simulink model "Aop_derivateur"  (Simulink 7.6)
settings: Solver=ode15s  StartTime=0.0  StopTime=1.4  RelTol=1e-3
InitFcn:
  | close all, clear all, clc
StopFcn:
  | close all, clc
  | load es.mat
  | plotyy(x(1,:),x(2,:),x(1,:),x(3,:))
  | title('montage dérivateur')
  | xlabel('temps')
  | grid
libraries: fl_lib x8, nesl_utility x3, simulink x1

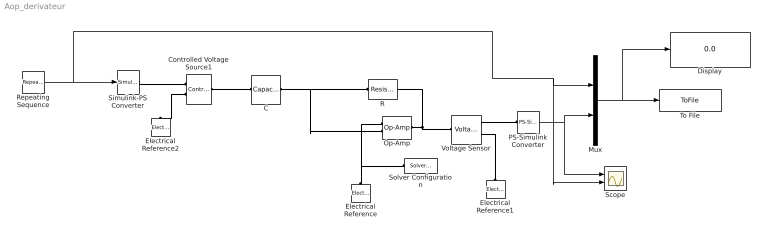
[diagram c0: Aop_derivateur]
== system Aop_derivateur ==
  C : fl_lib/Electrical/Electrical Elements/Capacitor  DialogController=NetworkEngine.DynNeDlgSource  SystemSampleTime=-1  c=100e-9 F  v0=0 V  r=1e-6 Ohm  g=0 1/Ohm  i_Log=off  v_Log=off  vc_Log=off  LocalVarNames=|current|voltage|power  LocalVarDescs=|Capacitor current (A)|Voltage across capacitor (V)|Power (W)  LocalVarLogging=[0 0 0]
  Controlled Voltage Source1 : fl_lib/Electrical/Electrical Sources/Controlled Voltage Source  DialogController=NetworkEngine.DynNeDlgSource  SystemSampleTime=-1  i_Log=off  v_Log=off  LocalVarNames=|current|voltage|power  LocalVarDescs=|Current (A)|Voltage (V)|Power (W)  LocalVarLogging=[0 0 0]
  Display : Display
  Electrical Reference : fl_lib/Electrical/Electrical Elements/Electrical Reference  DialogController=NetworkEngine.DynNeDlgSource  SystemSampleTime=-1  i_Log=off  LocalVarNames=|i  LocalVarDescs=|i  LocalVarLogging=[]
  Electrical Reference1 : fl_lib/Electrical/Electrical Elements/Electrical Reference  DialogController=NetworkEngine.DynNeDlgSource  SystemSampleTime=-1  i_Log=off  LocalVarNames=|i  LocalVarDescs=|i  LocalVarLogging=[]
  Electrical Reference2 : fl_lib/Electrical/Electrical Elements/Electrical Reference  DialogController=NetworkEngine.DynNeDlgSource  SystemSampleTime=-1  i_Log=off  LocalVarNames=|i  LocalVarDescs=|i  LocalVarLogging=[]
  Mux : Mux  Inputs=2
  Op-Amp : fl_lib/Electrical/Electrical Elements/Op-Amp  DialogController=NetworkEngine.DynNeDlgSource  SystemSampleTime=-1  i1_Log=off  v1_Log=off  outI_Log=off  LocalVarNames=|i1|v1|outI  LocalVarDescs=|i1|v1|outI  LocalVarLogging=[]
  PS-Simulink Converter : nesl_utility/PS-Simulink Converter  DialogController=NetworkEngine.DynNeUtilDlgSource  SystemSampleTime=-1  PhysicalDomain=network_engine_domain  LeftPortType=input  RightPortType=output  SubClassName=ps_output  Unit=1  AffineConversion=off
  R : fl_lib/Electrical/Electrical Elements/Resistor  DialogController=NetworkEngine.DynNeDlgSource  SystemSampleTime=-1  R=10e3 Ohm  i_Log=off  v_Log=off  LocalVarNames=|current|voltage|power  LocalVarDescs=|Resistor current (A)|Voltage across resistor (V)|Power (W)  LocalVarLogging=[0 0 0]
  Repeating Sequence : simulink/Sources/Repeating Sequence  SystemSampleTime=-1  rep_seq_t="[0  0.7 1.4 2.1 2.8 3.5 4.2 4.9]"  rep_seq_y="[0  0.1  0 .1 0  0.1  0 .1]"
  Scope : Scope  NumInputPorts=2
  Simulink-PS Converter : nesl_utility/Simulink-PS Converter  DialogController=NetworkEngine.DynNeUtilDlgSource  SystemSampleTime=-1  PhysicalDomain=network_engine_domain  LeftPortType=input  RightPortType=output  SubClassName=ps_input  Unit=1  AffineConversion=off  InputFilterTimeConstant=.001  UdotUserProvided=0
  Solver Configuration : nesl_utility/Solver Configuration  DialogController=NetworkEngine.DynNeUtilDlgSource  SystemSampleTime=-1  PhysicalDomain=network_engine_domain  LeftPortType=input  RightPortType=generic  SubClassName=solver  Accelerate=off  Profile=off  ResidualTolerance=1e-9  MaxNonlinIter=12  MaxModeIter=2  DoFixedCost=off  UseLocalSampling=off  DoDC=off  LinearAlgebra=Sparse  LocalSolverSampleTime=.001  LocalSolverChoice=NE_BACKWARD_EULER_ADVANCER  UseLocalSolver=off
  To File : ToFile  Filename=es.mat  MatrixName=x
  Voltage Sensor : fl_lib/Electrical/Electrical Sensors/Voltage Sensor  DialogController=NetworkEngine.DynNeDlgSource  SystemSampleTime=-1  i1_Log=off  v1_Log=off  LocalVarNames=|i1|v1  LocalVarDescs=|i1|v1  LocalVarLogging=[]
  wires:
  PS-Simulink Converter/1 -> Mux/2, Scope/1
  Mux/1 -> To File/1, Display/1
  Repeating Sequence/1 -> Simulink-PS Converter/1, Mux/1, Scope/2
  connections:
  Electrical Reference/LConn1 -- Op-Amp/LConn1 -- Solver Configuration/RConn1
  C/RConn1 -- R/LConn1 -- Op-Amp/LConn2
  Electrical Reference1/LConn1 -- Voltage Sensor/RConn2
  Voltage Sensor/RConn1 -- PS-Simulink Converter/LConn1
  Controlled Voltage Source1/RConn2 -- Electrical Reference2/LConn1
  Simulink-PS Converter/RConn1 -- Controlled Voltage Source1/RConn1
  C/LConn1 -- Controlled Voltage Source1/LConn1
  Op-Amp/RConn1 -- Voltage Sensor/LConn1 -- R/RConn1
